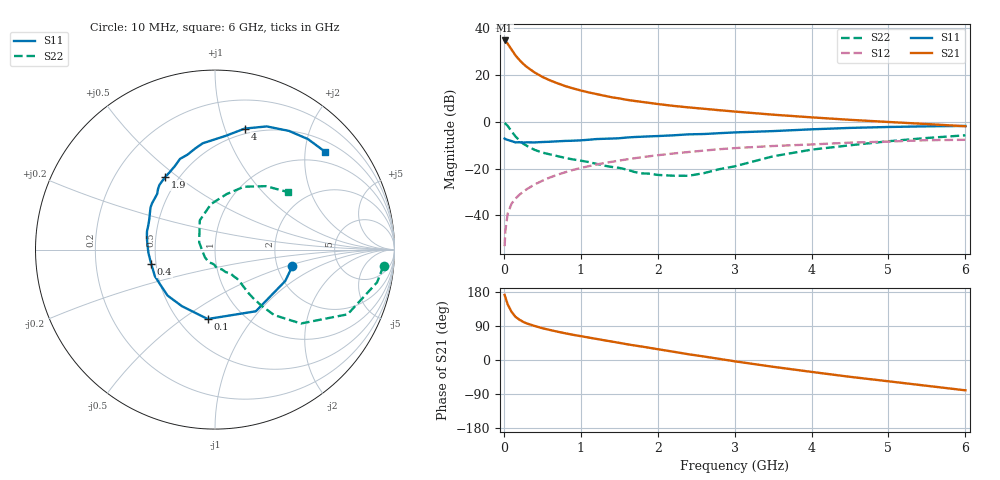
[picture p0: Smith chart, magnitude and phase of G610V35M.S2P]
! SIEMENS Small Signal Semiconductors
! BFG193
! Si NPN RF Bipolar Junction Transistor in SOT223
! VCE = 10 V  IC = 35 mA
! Common Emitter S-Parameters:  August  1996
# GHz  S  MA  R  50
!  f  S11  S21  S12  S22
! GHz  MAG  ANG  MAG  ANG  MAG  ANG  MAG  ANG
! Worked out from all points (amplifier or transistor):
!   36 points, 10 MHz to 6 GHz, reference 50 ohm
!   highest |S21| = 34.8 dB at 10 MHz (marker M1)
!   |S21| within 3 dB of that: start of sweep to 82.5 MHz
!   unconditionally stable (mu >= 1): 604.9 MHz to 2.496 GHz
!   at 250 MHz: K = 0.84, MSG = 27.4 dB, |S12| = -29.9 dB
!   at 1.4 GHz: K = 1.04, MAG = 12.6 dB, |S12| = -17.1 dB
!   at 6 GHz: K = 0.88, MSG = 2.9 dB, |S12| = -7.7 dB
!   S11 on the Smith chart (normalised r, x): 10 MHz: 2.42, -0.56; 100 MHz: 0.69, -0.63; 400 MHz: 0.47, -0.09; 1.9 GHz: 0.42, +0.45; 4 GHz: 0.45, +1.17; 6 GHz: 0.73, +2.44
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0.01  0.4408 -12.1  55.23 171.7  0.0022 89.2  0.9432 -5.5
0.02  0.4287 -24.1  53.53 165.5  0.0047 81.3  0.9214 -11.4
0.05  0.4121 -56.5  47.06 146.7  0.011 71.6  0.8223 -26.0
0.1  0.3888 -96.0  35.38 127.3  0.0178 66.0  0.6315 -40.7
0.15  0.3651 -120.4  26.68 114.2  0.0228 62.8  0.4917 -47.9
0.2  0.368 -135.9  21.35 106.7  0.0275 63.6  0.4081 -50.3
0.25  0.3621 -147.1  17.57 100.8  0.0319 63.7  0.3446 -51.8
0.3  0.3662 -156.1  14.92 96.4  0.0366 65.0  0.3074 -52.4
0.4  0.3643 -167.2  11.42 89.9  0.0459 65.6  0.2528 -52.4
0.5  0.3713 -177.0  9.198 83.9  0.0551 65.3  0.2211 -52.1
0.6  0.3767 176.3  7.736 79.2  0.0649 64.5  0.2019 -52.9
0.7  0.3846 170.7  6.669 74.6  0.0745 63.8  0.1851 -54.6
0.9  0.396 159.5  5.208 66.5  0.094 60.6  0.1577 -57.2
1.1  0.415 151.0  4.286 59.4  0.1126 57.8  0.1388 -64.6
1.4  0.4403 139.8  3.376 48.8  0.1398 51.9  0.1092 -76.9
1.9  0.4911 124.3  2.543 31.9  0.1851 41.5  0.0782 -113.2
2.2  0.5165 115.6  2.205 22.0  0.2108 34.6  0.0707 -142.8
3.5  0.6362 84.7  1.428 -17.9  0.3054 4.0  0.1839 117.4
4  0.6944 76.2  1.252 -31.4  0.3295 -5.6  0.2551 94.9
4.5  0.7444 67.2  1.108 -44.4  0.3601 -15.7  0.3163 78.1
5.5  0.8046 49.9  0.9 -68.1  0.4068 -38.8  0.4535 51.2
6  0.8206 41.6  0.808 -80.0  0.414 -52.2  0.5172 38.3
